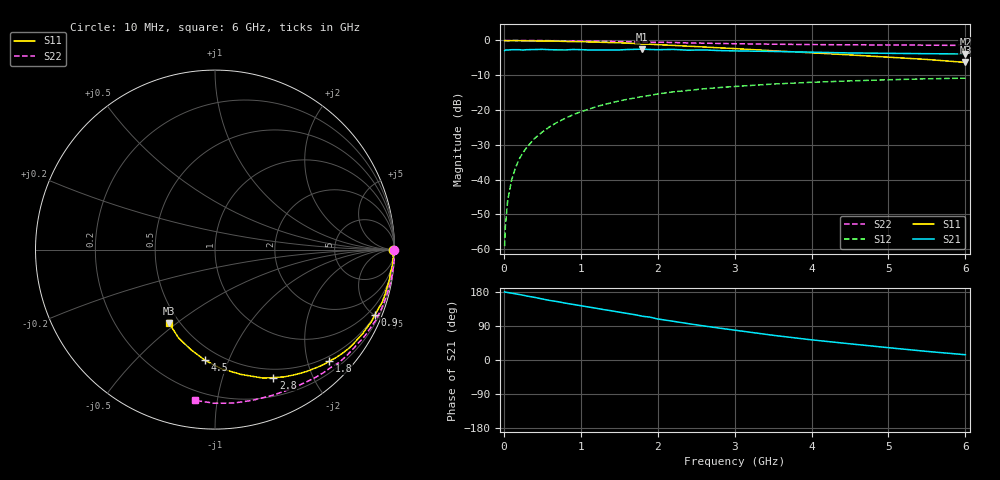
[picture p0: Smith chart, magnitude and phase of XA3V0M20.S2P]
! SIEMENS Discrete & RF Semiconductors
! BFY180
! Si NPN RF Bipolar Junction Transistor in MICRO-X
! VCE = 3 V  IC = 0.2 mA
! Common Emitter S-Parameters:  May  1997
# GHz  S  MA  R  50
!  f  S11  S21  S12  S22
! GHz  MAG  ANG  MAG  ANG  MAG  ANG  MAG  ANG
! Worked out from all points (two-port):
!   36 points, 10 MHz to 6 GHz, reference 50 ohm
!   highest |S21| = -2.51 dB at 1.8 GHz (marker M1); lowest = -3.9 dB at 6 GHz (marker M2)
!   |S21| within 3 dB of the highest: start of sweep to end of sweep
!   lowest |S11| = -6.3 dB at 6 GHz (marker M3), VSWR 2.87, Z = 22 - j23.5 ohm
!   |S11| at or under -10 dB: nowhere
!   |S22| runs from -1.4 to 0.0 dB; largest |S21 - S12| = 0.74
!   S11 on the Smith chart (normalised r, x): 10 MHz: open; 900 MHz: 0.51, -5.05; 1.8 GHz: 0.40, -2.40; 2.8 GHz: 0.40, -1.48; 4.5 GHz: 0.41, -0.83; 6 GHz: 0.44, -0.47
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0.01  0.9937 -0.2  0.712 179.9  0.0011 83.7  0.9999 -0.2
0.02  0.9927 -0.6  0.729 179.1  0.0021 88.2  0.9999 -0.4
0.05  0.989 -1.1  0.729 178.2  0.005 88.5  0.9997 -1.0
0.1  0.994 -2.4  0.736 176.5  0.0097 88.8  0.9996 -2.1
0.15  0.9918 -3.8  0.736 174.7  0.0146 88.7  0.9999 -3.0
0.2  0.9916 -4.9  0.736 172.9  0.0197 86.4  0.9994 -4.1
0.3  0.9858 -7.4  0.737 168.7  0.0292 84.0  0.9978 -6.0
0.4  0.986 -9.8  0.74 165.3  0.039 82.1  0.9974 -7.9
0.5  0.9813 -12.5  0.745 161.0  0.0482 79.4  0.996 -10.0
0.7  0.9768 -17.5  0.732 154.0  0.067 74.7  0.9909 -14.0
0.9  0.9622 -22.2  0.741 146.7  0.0854 70.4  0.9863 -17.9
1.1  0.952 -27.0  0.73 139.9  0.1026 66.3  0.9799 -21.8
1.4  0.9326 -34.4  0.727 129.9  0.1271 59.9  0.9678 -27.7
1.8  0.8895 -44.3  0.749 115.5  0.156 52.1  0.9497 -35.0
2.2  0.8496 -53.1  0.743 102.2  0.1821 44.3  0.9351 -42.2
2.6  0.8063 -61.6  0.731 89.9  0.2016 37.5  0.9141 -48.6
2.8  0.7837 -65.5  0.715 84.2  0.2101 34.3  0.9059 -51.7
3.5  0.71 -78.3  0.695 65.2  0.236 24.3  0.8832 -61.9
4  0.6647 -86.9  0.678 53.2  0.2503 17.5  0.8723 -68.9
4.5  0.6197 -95.1  0.661 42.7  0.2619 11.4  0.8654 -76.1
5.5  0.533 -112.3  0.645 22.7  0.2808 -0.4  0.8558 -90.4
6  0.4833 -122.0  0.639 13.9  0.287 -6.4  0.8474 -97.6
